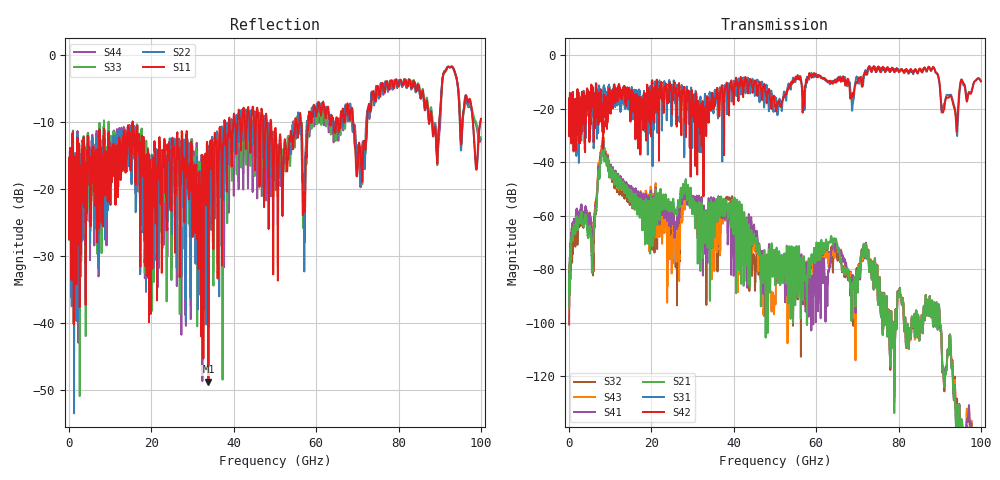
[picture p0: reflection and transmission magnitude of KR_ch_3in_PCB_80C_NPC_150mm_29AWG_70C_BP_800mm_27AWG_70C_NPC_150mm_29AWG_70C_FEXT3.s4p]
# GHz S RI R 45
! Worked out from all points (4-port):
!   4000 points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, 25 MHz to 100 GHz, reference 45 ohm
!   strongest paths, dB at 25 MHz, 25.02 GHz, 50.02 GHz, 75.03 GHz, 100 GHz:
!     S42: -21.8, -20.6, -18.8, -4.2, -9.7
!     S31: -21.8, -12.9, -15.6, -4.9, -9.6
!     S21: -94.3, -57.6, -84.6, -92.8, -155.0
!     S41: -94.2, -60.7, -78.5, -92.7, -150.1
!     S43: -94.3, -73.9, -91.6, -92.4, -159.4
!     S32: -100.8, -72.8, -84.3, -92.6, -157.2
!   lowest |S11| = -48.8 dB at 33.85 GHz (marker M1), VSWR 1.01, Z = 45.3 - j0.0686 ohm
!   |S11| at or under -10 dB: start of sweep to 15.45 GHz; 15.46 GHz to 37.71 GHz (22.25 GHz wide, 83.7 % of centre); 49.07 GHz to 54.91 GHz (5.843 GHz wide, 11.2 % of centre)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
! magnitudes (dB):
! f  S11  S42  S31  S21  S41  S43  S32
! 25 MHz  -17.2  -21.8  -21.8  -94.3  -94.2  -94.3  -100.8
! 5.775 GHz  -17.0  -14.4  -18.6  -73.8  -68.3  -69.5  -73.8
! 8.3 GHz  -16.1  -27.3  -14.6  -33.5  -31.9  -30.7  -32.1
! 24.73 GHz  -18.3  -11.7  -14.2  -54.9  -58.8  -69.4  -64.4
! 28.7 GHz  -14.0  -12.7  -14.7  -54.3  -55.8  -56.0  -54.6
! 33.85 GHz  -48.8  -24.0  -21.9  -56.9  -54.8  -56.1  -58.8
! 100 GHz  -9.5  -9.7  -9.6  -155.0  -150.1  -159.4  -157.2
